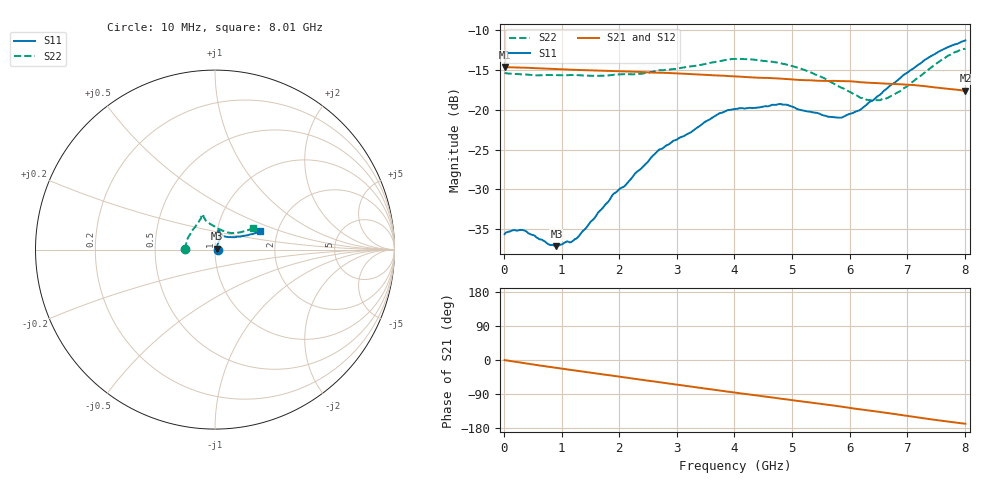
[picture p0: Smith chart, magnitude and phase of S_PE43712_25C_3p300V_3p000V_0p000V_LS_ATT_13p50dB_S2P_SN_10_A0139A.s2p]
! DEVICE ID: PE43712
! File Path: z:\PE43713\PE43713_CHAR_NOM_04292014\AMB\3p300\LS_ATT_13p50dB\PE43713_AMB_3p300V_3p000V_0p000V_LS_ATT_13p50dB_S2P_SN_10_A0139A.s2p
! Serial: 10
! Lot: A0139A
! Temp: 25C
! VDD: 3.300
! VSS: 0.000
! Control_Hi: 3.000
! Control_Lo: 0.000
! Attenuation Step: 13.50dB
! Port 1: RF1
! Port 2: RF2
! ThroughPath:1-2
! IDD: 0.0001473272
! ISS: -8.97e-008
#  Hz  S  RI  R  50
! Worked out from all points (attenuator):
!   801 points, 10 MHz to 8.01 GHz, reference 50 ohm
!   highest |S21| = -14.69 dB at 10 MHz (marker M1); lowest = -17.7 dB at 8.01 GHz (marker M2)
!   lowest |S11| = -37.1 dB at 910 MHz (marker M3), VSWR 1.03, Z = 51.3 + j0.587 ohm
!   |S11| at or under -10 dB: start of sweep to end of sweep
!   |S22| runs from -18.9 to -12.4 dB; largest |S21 - S12| = 0.00066
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1e7  0.0166 0.000306  0.1843 -0.000939  0.1844 -0.000916  -0.1693 0.00108
3.3e8  0.0176 0.000519  0.181 -0.0252  0.1808 -0.025  -0.1649 0.0195
7.8e8  0.0137 0.00409  0.1713 -0.0557  0.1713 -0.0558  -0.1586 0.0436
9.1e8  0.0127 0.00573  0.1675 -0.0639  0.1676 -0.0639  -0.1565 0.0502
1.18e9  0.011 0.0101  0.1588 -0.0795  0.1587 -0.0796  -0.1512 0.0646
1.35e9  0.0112 0.0129  0.1528 -0.0889  0.1528 -0.0889  -0.1468 0.0723
1.9e9  0.0137 0.0263  0.1299 -0.1161  0.1299 -0.116  -0.1296 0.1024
2.11e9  0.0149 0.0302  0.1199 -0.1251  0.12 -0.125  -0.1237 0.1114
2.68e9  0.0233 0.0507  0.0897 -0.1443  0.0896 -0.1443  -0.099 0.1455
3.72e9  0.0241 0.0906  0.0284 -0.1609  0.0283 -0.1608  -0.0759 0.1854
4.01e9  0.0228 0.0983  0.0113 -0.161  0.0113 -0.161  -0.0759 0.1933
4.79e9  0.0207 0.1064  -0.0319 -0.1531  -0.0319 -0.1533  -0.065 0.1846
5.35e9  0.0309 0.0911  -0.0592 -0.1404  -0.0591 -0.1403  -0.051 0.1617
5.64e9  0.041 0.0803  -0.0719 -0.133  -0.0719 -0.133  -0.033 0.1475
5.88e9  0.0515 0.0734  -0.0834 -0.1256  -0.0832 -0.1256  -0.0141 0.1354
6.17e9  0.0702 0.0699  -0.0954 -0.1138  -0.0951 -0.1139  0.0138 0.1186
6.38e9  0.0887 0.0703  -0.1022 -0.1054  -0.102 -0.1054  0.0367 0.1076
6.68e9  0.1199 0.0705  -0.1117 -0.0924  -0.1115 -0.0925  0.072 0.0954
6.99e9  0.1514 0.0753  -0.1203 -0.0777  -0.1201 -0.0777  0.1044 0.092
7.37e9  0.194 0.0842  -0.1267 -0.0575  -0.1266 -0.0574  0.1484 0.0985
7.72e9  0.2285 0.0937  -0.1286 -0.04  -0.1285 -0.0401  0.1882 0.1104
8.01e9  0.2496 0.105  -0.1282 -0.0269  -0.128 -0.0271  0.2092 0.1182
